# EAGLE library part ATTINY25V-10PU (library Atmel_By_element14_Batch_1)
8-bit Microcontroller with 2/4/8KBytes In-System Programmable Flash
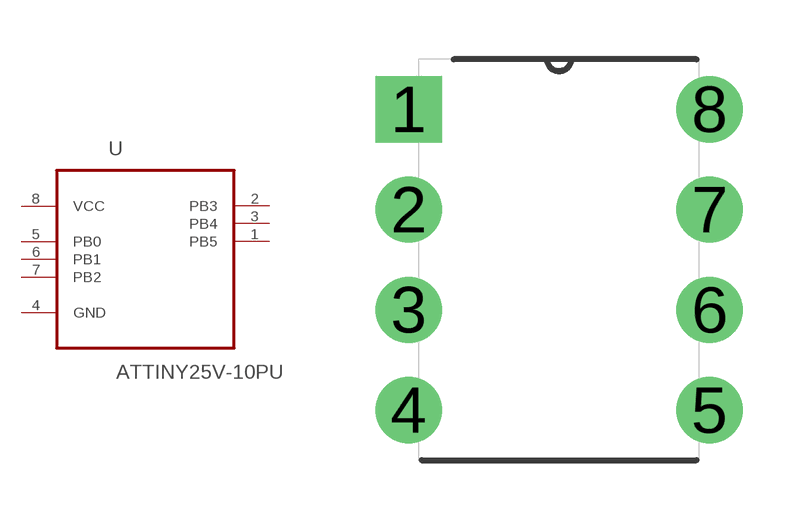
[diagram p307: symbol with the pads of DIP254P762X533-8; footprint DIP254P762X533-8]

Designator prefix U

## ATTINY25V-10PU (MPN: ATTINY25V-10PU; OC_FARNELL: 1455144; OC_NEWARK: 58M3780; PACKAGE: PDIP-8; SUPPLIER: Atmel)  [DIP254P762X533-8]
1  PB5
2  PB3
3  PB4
4  GND  pas
5  PB0
6  PB1
7  PB2
8  VCC  pwr

## Footprint DIP254P762X533-8 (pad centres in mm)
drill 1.118 square: 1 -7.62,7.62
drill 1.118: 2 -7.62,5.08; 3 -7.62,2.54; 4 -7.62,0; 5 0,0; 6 0,2.54; 7 0,5.08; 8 0,7.62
